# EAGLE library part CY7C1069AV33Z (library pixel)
2M x 8 Static RAM Source: CYPRESS cy7c1069av33_8.pdf
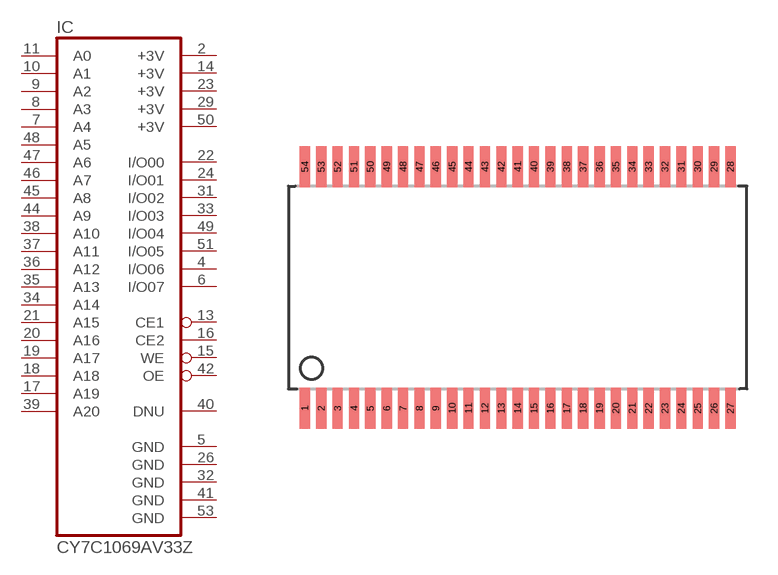
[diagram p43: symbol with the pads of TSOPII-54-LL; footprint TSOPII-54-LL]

Designator prefix IC

## CY7C1069AV33Z  [TSOPII-54-LL]
2  +3V  pwr
4  I/O06
5  GND  pwr
6  I/O07
7  A4  in
8  A3  in
9  A2  in
10  A1  in
11  A0  in
13  CE1  in
14  +3V  pwr
15  WE  in
16  CE2  in
17  A19  in
18  A18  in
19  A17  in
20  A16  in
21  A15  in
22  I/O00
23  +3V  pwr
24  I/O01
26  GND  pwr
29  +3V  pwr
31  I/O02
32  GND  pwr
33  I/O03
34  A14  in
35  A13  in
36  A12  in
37  A11  in
38  A10  in
39  A20  in
40  DNU  pas
41  GND  pwr
42  OE  in
44  A9  in
45  A8  in
46  A7  in
47  A6  in
48  A5  in
49  I/O04
50  +3V  pwr
51  I/O05
53  GND  pwr

## Footprint TSOPII-54-LL (pad centres in mm)
54-pin TSOP II (51-85160) Source: CYPRESS cy7c1069av33_8.pdf
smd 0.5 x 2: 1 -10.4,-5.9; 2 -9.6,-5.9; 3 -8.8,-5.9; 4 -8,-5.9; 5 -7.2,-5.9; 6 -6.4,-5.9; 7 -5.6,-5.9; 8 -4.8,-5.9; 9 -4,-5.9; 10 -3.2,-5.9; 11 -2.4,-5.9; 12 -1.6,-5.9; 13 -0.8,-5.9; 14 0,-5.9; 15 0.8,-5.9; 16 1.6,-5.9; 17 2.4,-5.9; 18 3.2,-5.9; 19 4,-5.9; 20 4.8,-5.9; 21 5.6,-5.9; 22 6.4,-5.9; 23 7.2,-5.9; 24 8,-5.9; 25 8.8,-5.9; 26 9.6,-5.9; 27 10.4,-5.9; 28 10.4,5.9; 29 9.6,5.9; 30 8.8,5.9; 31 8,5.9; 32 7.2,5.9; 33 6.4,5.9; 34 5.6,5.9; 35 4.8,5.9; 36 4,5.9; 37 3.2,5.9; 38 2.4,5.9; 39 1.6,5.9; 40 0.8,5.9; 41 0,5.9; 42 -0.8,5.9; 43 -1.6,5.9; 44 -2.4,5.9; 45 -3.2,5.9; 46 -4,5.9; 47 -4.8,5.9; 48 -5.6,5.9; 49 -6.4,5.9; 50 -7.2,5.9; 51 -8,5.9; 52 -8.8,5.9; 53 -9.6,5.9; 54 -10.4,5.9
